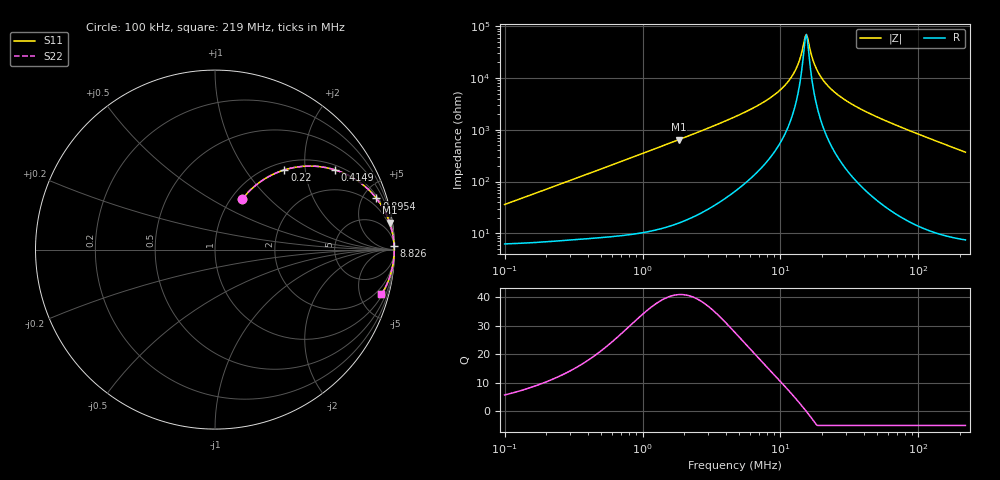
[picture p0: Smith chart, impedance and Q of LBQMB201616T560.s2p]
! LBQMB201616T560  S-PARAMETER MODEL  ( General Type )
! Model Generated by TAIYO YUDEN Corporation (http://www.ty-top.com)
! Version 1.0
! TAIYO YUDEN Control No. 191025NI43SB-FBB
! Copyright(c) 2019 TAIYO YUDEN CO.,LTD. All Rights Reserved.
! Product Description (link to TY-COMPAS)
! https://ds.yuden.co.jp/TYCOMPAS/or/detail?pn=LBQMB201616T560J&u=M
! Products Name : Inductors
! Characteristics :
!  Inductance : 56 uH , SRF(min) : 12 MHz , DC Resistance(max) : 7.67 Ohm , Rated Current : 95 mA
!  Case Size : 2.0 x 1.6 / 0.079 x 0.063 [mm/inch] , Thickness : 1.6 / 0.063 [mm/inch]
!  (Conditions: Temperature = 25 degC , DC Bias Current/Voltage = 0A / 0V)
! External Node Assignments :
!  1  o---GGG---o  2
! GND o---------o GND
! Frequency Range : 0.1MHz  -  218.972167MHz  [ 402 STEP ]
# MHz S RI R 50
! Freq[MHz].  S11 Real  S11 Imag  S21 Real  S21 Imag  S12 Real  S12 Imag  S22 Real  S22 Imag
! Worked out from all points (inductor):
!   401 points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, 100 kHz to 219 MHz, reference 50 ohm
!   read as one part in series: L = 56.3 uH near 103.9 kHz
!   highest Q = 40.9 at 1.824 MHz (marker M1), where L = 56 uH
!   self-resonance near 15.12 MHz
!   S11 on the Smith chart (normalised r, x): 100 kHz: 1.12, +0.71; 220 kHz: 1.14, +1.55; 414.9 kHz: 1.16, +2.90; 895.4 kHz: 1.20, +6.24; 8.826 MHz: 8, +90; 219 MHz: 1.15, -7.38
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0.1  0.1529 0.2827  0.8471 -0.2827  0.8471 -0.2827  0.1529 0.2827
0.146899  0.2414 0.3698  0.7586 -0.3698  0.7586 -0.3698  0.2414 0.3698
0.219983  0.3865 0.444  0.6135 -0.444  0.6135 -0.444  0.3865 0.444
0.362673  0.6112 0.4581  0.3888 -0.4581  0.3888 -0.4581  0.6112 0.4581
0.414927  0.6697 0.4438  0.3303 -0.4438  0.3303 -0.4438  0.6697 0.4438
0.895387  0.8997 0.2851  0.1003 -0.2851  0.1003 -0.2851  0.8997 0.2851
1.315317  0.95 0.2053  0.05 -0.2053  0.05 -0.2053  0.95 0.2053
1.823882  0.9728 0.151  0.0272 -0.151  0.0272 -0.151  0.9728 0.151
4.770297  0.995 0.0543  0.00498 -0.0543  0.00498 -0.0543  0.995 0.0543
8.826256  0.9979 0.0219  0.00215 -0.0219  0.00215 -0.0219  0.9979 0.0219
10.6976  0.9982 0.0139  0.00177 -0.0139  0.00177 -0.0139  0.9982 0.0139
12.47654  0.9984 0.00791  0.00157 -0.00791  0.00157 -0.00791  0.9984 0.00791
13.73564  0.9985 0.00424  0.00149 -0.00424  0.00149 -0.00424  0.9985 0.00424
15.12181  0.9986 0.000601  0.00144 -0.000601  0.00144 -0.000601  0.9986 0.000601
15.71469  0.9986 -0.000853  0.00142 0.000853  0.00142 0.000853  0.9986 -0.000853
16.97108  0.9986 -0.00377  0.00141 0.00377  0.00141 0.00377  0.9986 -0.00377
17.97887  0.9986 -0.00598  0.00142 0.00598  0.00142 0.00598  0.9986 -0.00598
19.79326  0.9986 -0.00971  0.00145 0.00971  0.00145 0.00971  0.9986 -0.00971
24.93039  0.9983 -0.0191  0.00167 0.0191  0.00167 0.0191  0.9983 -0.0191
35.92506  0.9974 -0.0363  0.00261 0.0363  0.00261 0.0363  0.9974 -0.0363
61.54953  0.9934 -0.0712  0.00656 0.0712  0.00656 0.0712  0.9934 -0.0712
218.9722  0.9272 -0.2499  0.0728 0.2499  0.0728 0.2499  0.9272 -0.2499
